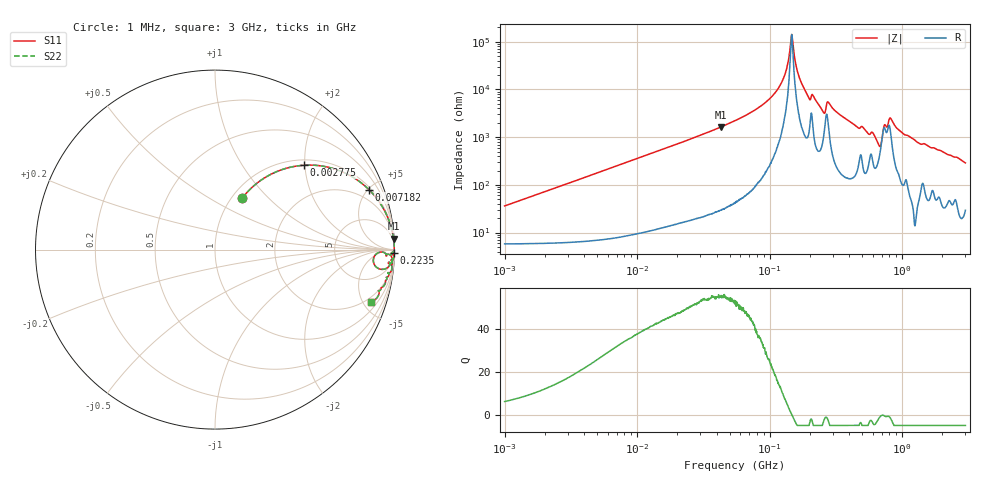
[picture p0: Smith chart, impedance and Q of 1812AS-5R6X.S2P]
!s-Parameter Generated by FASTRON Sdn. Bhd.
!FASTRON P/N : 1812AS-5R6X
!Keysight Technologies,E4991B,MY54100416,A.01.15
!Date created: Fri Oct 13 16:03:24 2023
!Version  : Rev00 Fri Oct 13 16:03:24 2023
!Data & Calibration Information:
!Freq	S11	S21	S12	S22
!PortZ  Port1:50+j0  Port2:50+j0
!When reading, reference impedance value at option line is always used.
! Remarks : This data is being provided solely for informational purposes.
# Hz S dB R 50
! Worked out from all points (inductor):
!   1601 points, 1 MHz to 3 GHz, reference 50 ohm
!   read as one part in series: L = 5.67 uH near 1.041 MHz
!   highest Q = 55.2 at 43.08 MHz (marker M1), where L = 6.07 uH
!   self-resonance near 146.8 MHz
!   S11 on the Smith chart (normalised r, x): 1 MHz: 1.12, +0.71; 2.775 MHz: 1.12, +1.97; 7.182 MHz: 1.16, +5.10; 223.5 MHz: open; 3 GHz: 1.59, -5.74
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1000000  -9.80 62.2  -0.96 -18.6  -0.96 -18.6  -9.80 62.2
2775447  -3.32 43.5  -3.23 -42.9  -3.23 -42.9  -3.32 43.5
3804036  -2.08 35.5  -4.72 -51.8  -4.72 -51.8  -2.08 35.5
7181929  -0.71 21.1  -8.85 -67.1  -8.85 -67.1  -0.71 21.1
1.447069e7  -0.20 10.9  -14.44 -77.7  -14.44 -77.7  -0.20 10.9
4.307715e7  -0.03 3.5  -24.34 -85.5  -24.34 -85.5  -0.03 3.5
5.477226e7  -0.02 2.6  -26.91 -86.3  -26.91 -86.3  -0.02 2.6
1.120285e8  -0.01 0.6  -39.18 -86.1  -39.18 -86.1  -0.01 0.6
1.30174e8  -0.01 0.3  -46.17 -82.2  -46.17 -82.2  -0.01 0.3
1.467848e8  -0.01 0.0  -63.07 -3.0  -63.07 -3.0  -0.01 0.0
1.7056e8  -0.01 -0.4  -43.83 82.1  -43.83 82.1  -0.01 -0.4
1.952332e8  -0.02 -0.8  -37.11 80.8  -37.11 80.8  -0.02 -0.8
2.083556e8  -0.04 -0.7  -37.89 67.6  -37.89 67.6  -0.04 -0.7
2.234756e8  -0.02 -1.0  -35.35 82.9  -35.35 82.9  -0.02 -1.0
2.519921e8  -0.06 -1.6  -30.89 75.0  -30.89 75.0  -0.06 -1.6
2.813178e8  -0.04 -1.1  -34.18 75.3  -34.18 75.3  -0.04 -1.1
4.570858e8  -0.08 -3.4  -24.36 79.8  -24.36 79.8  -0.08 -3.4
6.018993e8  -0.20 -4.4  -21.95 71.6  -21.95 71.6  -0.20 -4.4
6.685918e8  -0.73 -6.7  -17.24 50.9  -17.24 50.9  -0.73 -6.7
7.925923e8  -0.31 -1.5  -27.25 35.8  -27.25 35.8  -0.31 -1.5
1.333714e9  -0.14 -7.5  -17.68 79.1  -17.68 79.1  -0.14 -7.5
3e9  -0.76 -18.4  -9.95 65.7  -9.95 65.7  -0.76 -18.4
